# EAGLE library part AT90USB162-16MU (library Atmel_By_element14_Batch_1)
Microcontroller
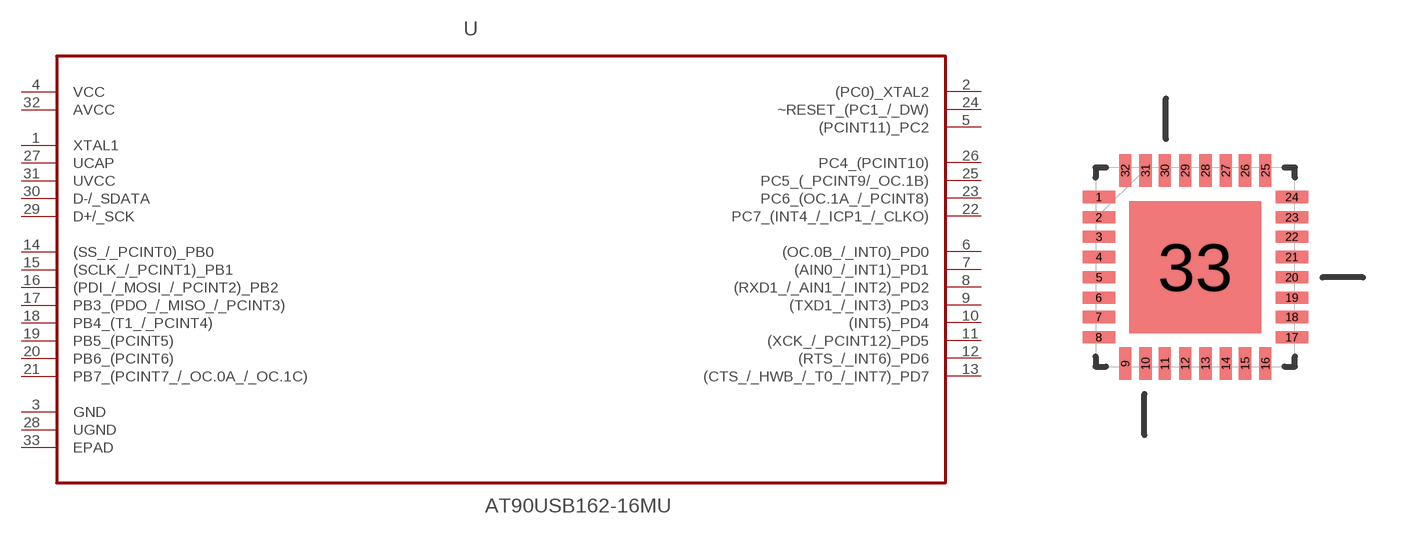
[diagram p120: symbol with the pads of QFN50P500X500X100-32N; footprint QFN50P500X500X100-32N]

Designator prefix U

## AT90USB162-16MU (DESCRIPTION: Microcontroller; MPN: AT90USB162-16MU; OC_FARNELL: 1455074; OC_NEWARK: 58M3869; PACKAGE: QFN-32; SUPPLIER: ATMEL)  [QFN50P500X500X100-32N]
1  XTAL1  in
2  (PC0)_XTAL2
3  GND  pas
4  VCC  pwr
5  (PCINT11)_PC2
6  (OC.0B_/_INT0)_PD0
7  (AIN0_/_INT1)_PD1
8  (RXD1_/_AIN1_/_INT2)_PD2
9  (TXD1_/_INT3)_PD3
10  (INT5)_PD4
11  (XCK_/_PCINT12)_PD5
12  (RTS_/_INT6)_PD6
13  (CTS_/_HWB_/_T0_/_INT7)_PD7
14  (SS_/_PCINT0)_PB0
15  (SCLK_/_PCINT1)_PB1
16  (PDI_/_MOSI_/_PCINT2)_PB2
17  PB3_(PDO_/_MISO_/_PCINT3)
18  PB4_(T1_/_PCINT4)
19  PB5_(PCINT5)
20  PB6_(PCINT6)
21  PB7_(PCINT7_/_OC.0A_/_OC.1C)
22  PC7_(INT4_/_ICP1_/_CLKO)
23  PC6_(OC.1A_/_PCINT8)
24  ~RESET_(PC1_/_DW)
25  PC5_(_PCINT9/_OC.1B)
26  PC4_(PCINT10)
27  UCAP  in
28  UGND  pas
29  D+/_SCK  in
30  D-/_SDATA  in
31  UVCC  pwr
32  AVCC  pwr
33  EPAD  pas

## Footprint QFN50P500X500X100-32N (pad centres in mm)
smd 0.813 x 0.305: 1 -2.413,1.753; 2 -2.413,1.245; 3 -2.413,0.762; 4 -2.413,0.254; 5 -2.413,-0.254; 6 -2.413,-0.762; 7 -2.413,-1.245; 8 -2.413,-1.753; 17 2.413,-1.753; 18 2.413,-1.245; 19 2.413,-0.762; 20 2.413,-0.254; 21 2.413,0.254; 22 2.413,0.762; 23 2.413,1.245; 24 2.413,1.753
smd 0.305 x 0.813: 9 -1.753,-2.413; 10 -1.245,-2.413; 11 -0.762,-2.413; 12 -0.254,-2.413; 13 0.254,-2.413; 14 0.762,-2.413; 15 1.245,-2.413; 16 1.753,-2.413; 25 1.753,2.413; 26 1.245,2.413; 27 0.762,2.413; 28 0.254,2.413; 29 -0.254,2.413; 30 -0.762,2.413; 31 -1.245,2.413; 32 -1.753,2.413
smd 3.302 x 3.302: 33 0,0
